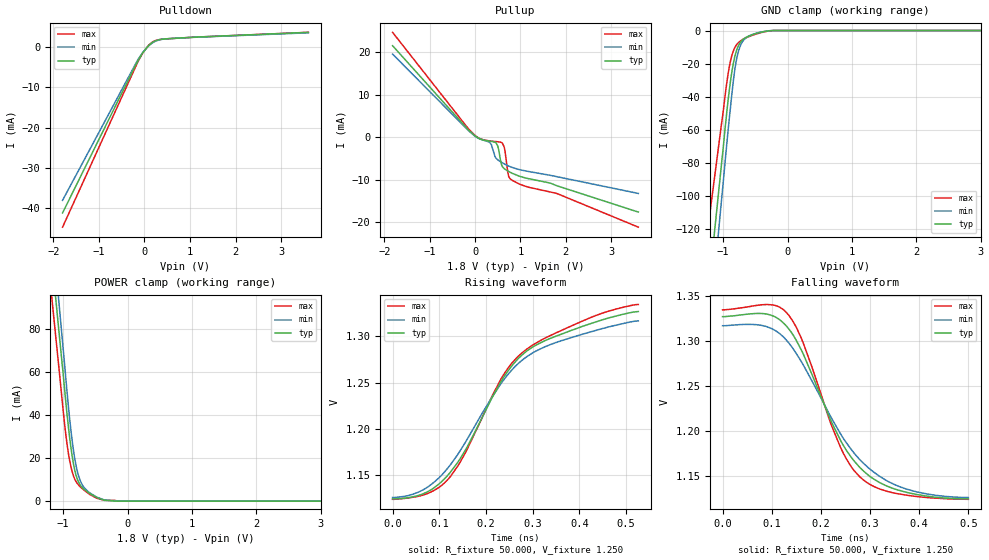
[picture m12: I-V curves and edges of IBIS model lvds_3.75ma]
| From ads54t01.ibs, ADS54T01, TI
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[Model]   lvds_3.75ma
Model_type 3-state
Vref=1.250E+00
Rref=5.000E+01
Cref=0.000E+00
Vmeas=1.250E+00
C_comp   7.860E-13   7.790E-13   7.930E-13
[Voltage Range]   1.800E+00   1.650E+00   1.950E+00
[POWER Clamp Reference]   1.800E+00   1.650E+00   1.950E+00
[GND Clamp Reference]   0.000E+00   0.000E+00   0.000E+00
[Pullup Reference]   1.800E+00   1.650E+00   1.950E+00
[Pulldown Reference]   0.000E+00   0.000E+00   0.000E+00
[Temperature Range]   25   85   -40
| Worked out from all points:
|   slope of the pulldown table from 0 to 0.27 V, typ, clamps not added: 106 ohm
|   slope of the pullup table from 0 to 0.27 V, typ, clamps not added: 231 ohm
|   GND clamp passes 1 mA (typ) near -0.41 V on its own axis
|   POWER clamp passes 1 mA (typ) near -0.41 V on its own axis
|   rising waveform, R_fixture 50.000, V_fixture 1.250: 20-80 % time 153ps typ, 161ps min, 159ps max; typ from 1.12 V to 1.33 V
|   falling waveform, R_fixture 50.000, V_fixture 1.250: 20-80 % time 107ps typ, 128ps min, 87.5ps max; typ from 1.33 V to 1.12 V
[GND Clamp]
-1.8V     -374.4mA   -423.5mA   -288.4mA
-1.02V    -78.69mA   -100.5mA   -54.92mA
-920mV    -41.17mA   -59.34mA   -25.51mA
-860mV    -23.88mA   -36.88mA   -14.48mA
-820mV    -15.94mA   -23.97mA   -10.43mA
-780mV    -10.76mA   -15.27mA   -8.038mA
-740mV    -7.589mA   -9.923mA   -6.562mA
-700mV    -5.657mA   -6.755mA   -5.499mA
-640mV    -4.069mA   -4.329mA   -4.359mA
-460mV    -1.489mA   -1.354mA   -1.806mA
-220mV    -4.201uA   -14.01uA   -11.29uA
3.6V      0A         0A         0A
[Power Clamp]
-1.8V     302.8mA    334.3mA    279.3mA
-1.76V    290.6mA    320.1mA    266.6mA
-1.06V    77.25mA    90.47mA    60.21mA
-940mV    40.5mA     50.88mA    26.54mA
-880mV    24.97mA    33.1mA     16.1mA
-820mV    14.43mA    19.78mA    10.24mA
-780mV    10.23mA    13.83mA    8.195mA
-720mV    6.913mA    8.542mA    6.262mA
-580mV    3.451mA    3.702mA    2.982mA
-360mV    441.4uA    538.8uA    356.5uA
-140mV    0A         9.789uA    18.55uA
3.6V      0A         0A         0A
[Pullup]
-1.82V    21.56mA    19.59mA    24.7mA
-20mV     502.5uA    417.3uA    621.4uA
320mV     -908.4uA   -1.135mA   -843.6uA
460mV     -1.284mA   -4.894mA   -999.4uA
500mV     -2.055mA   -5.282mA   -1.042mA
600mV     -6.878mA   -5.978mA   -1.361mA
660mV     -7.502mA   -6.338mA   -3.209mA
740mV     -8.02mA    -6.749mA   -9.136mA
780mV     -8.251mA   -6.927mA   -9.822mA
1.16V     -9.686mA   -8.001mA   -11.7mA
1.8V      -11.38mA   -9.245mA   -13.19mA
3.6V      -17.58mA   -13.2mA    -21.13mA
[Pulldown]
-1.8V     -41.19mA   -38.05mA   -44.73mA
-160mV    -3.661mA   -3.396mA   -3.976mA
-40mV     -1.393mA   -1.32mA    -1.475mA
80mV      280.3uA    221.6uA    367.5uA
180mV     1.23mA     1.129mA    1.343mA
320mV     1.869mA    1.817mA    1.891mA
520mV     2.131mA    2.128mA    2.103mA
3.6V      3.697mA    3.587mA    3.708mA
[Rising Waveform]
R_fixture = 50.000
V_fixture = 1.250
V_fixture_min = 1.250
V_fixture_max = 1.250
|  time   V(typ)   V(min)   V(max)
0s        1.124V     1.126V     1.124V
66ps      1.13V      1.134V     1.129V
120ps     1.151V     1.159V     1.146V
156ps     1.177V     1.186V     1.174V
234ps     1.253V     1.25V      1.256V
260ps     1.271V     1.266V     1.274V
288ps     1.284V     1.278V     1.286V
338ps     1.298V     1.291V     1.301V
426ps     1.314V     1.305V     1.321V
526ps     1.327V     1.317V     1.335V
[Falling Waveform]
R_fixture = 50.000
V_fixture = 1.250
V_fixture_min = 1.250
V_fixture_max = 1.250
|  time   V(typ)   V(min)   V(max)
0s        1.327V     1.317V     1.335V
86ps      1.33V      1.316V     1.34V
112ps     1.325V     1.31V      1.338V
134ps     1.314V     1.298V     1.329V
164ps     1.286V     1.273V     1.298V
240ps     1.189V     1.197V     1.181V
264ps     1.169V     1.178V     1.158V
288ps     1.155V     1.163V     1.145V
372ps     1.132V     1.136V     1.129V
500ps     1.124V     1.126V     1.124V
[Ramp]
dV/dt_r   1.1216E-01/1.5250E-10   1.1460E-01/1.6090E-10   1.2642E-01/1.5850E-10
dV/dt_f   1.1216E-01/1.0691E-10   1.1460E-01/1.2806E-10   1.2642E-01/8.7078E-11
R_load = 50
